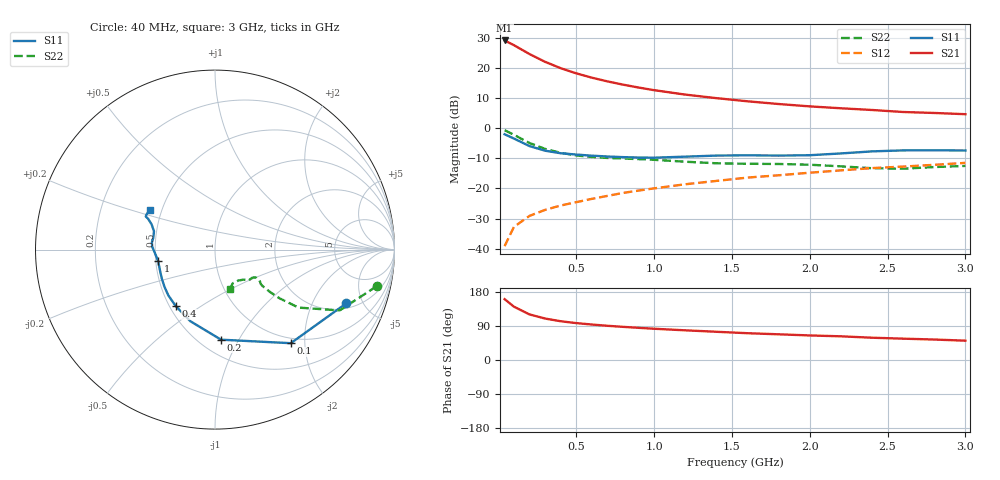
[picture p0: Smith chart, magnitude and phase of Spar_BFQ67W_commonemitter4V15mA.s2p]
! Filename:  BFQ67WD.S2P  Version:  4.0
! NXP part #: BFQ67W  Date: Jun 1994
! Bias condition: Vce=4V, Ic=15mA
#  MHz  S  MA  R  50
! Freq  S11  S21  S12  S22  !GUM [dB]
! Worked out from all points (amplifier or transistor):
!   21 points, 40 MHz to 3 GHz, reference 50 ohm
!   highest |S21| = 29.1 dB at 40 MHz (marker M1)
!   |S21| within 3 dB of that: start of sweep to 148.6 MHz
!   unconditionally stable (mu >= 1): 677.7 MHz to end of sweep
!   at 300 MHz: K = 0.73, MSG = 24.6 dB, |S12| = -27.1 dB
!   at 1 GHz: K = 1.07, MAG = 14.6 dB, |S12| = -20.0 dB
!   at 3 GHz: K = 1.01, MAG = 7.5 dB, |S12| = -11.5 dB
!   lowest NFmin = 1.95 dB at 1 GHz
!   S11 on the Smith chart (normalised r, x): 40 MHz: 2.32, -3.69; 100 MHz: 0.91, -1.72; 200 MHz: 0.63, -0.85; 400 MHz: 0.54, -0.40; 1 GHz: 0.52, -0.07; 3 GHz: 0.43, +0.23
40  0.79 -22.3  28.45 160.6  0.011 77.9  0.923 -12.8
100  0.671 -51.0  23.73 140.7  0.023 66.3  0.773 -26.0
200  0.503 -86.2  16.93 120.3  0.035 59.3  0.566 -34.8
300  0.422 -109.0  12.58 109.4  0.044 59.2  0.452 -37.0
400  0.383 -124.9  9.869 102.3  0.052 61.1  0.389 -37.6
500  0.364 -135.7  8.104 97.4  0.059 62.9  0.352 -37.6
600  0.349 -144.0  6.867 93.6  0.067 64.4  0.332 -37.4
700  0.338 -151.0  5.962 90.3  0.075 66.2  0.32 -37.0
800  0.33 -157.1  5.263 87.5  0.084 67.7  0.313 -36.1
900  0.325 -163.0  4.713 84.9  0.092 68.6  0.306 -35.2
1000  0.323 -168.5  4.261 82.5  0.1 69.3  0.298 -34.5
1200  0.336 -177.1  3.598 78.3  0.117 70.4  0.277 -34.2
1400  0.35 177.6  3.142 74.5  0.133 71.3  0.261 -36.6
1600  0.354 173.6  2.785 70.7  0.151 71.1  0.256 -40.7
1800  0.35 169.2  2.51 67.8  0.165 71.7  0.254 -43.0
2000  0.355 163.3  2.293 64.8  0.182 71.9  0.247 -43.9
2200  0.38 158.3  2.133 62.5  0.199 72.5  0.232 -46.0
2400  0.411 155.2  1.998 58.8  0.217 72.1  0.216 -53.0
2600  0.427 154.5  1.85 56.3  0.23 71.4  0.212 -62.0
2800  0.429 153.1  1.783 54.0  0.246 71.7  0.226 -67.3
3000  0.425 149.1  1.701 51.0  0.265 71.2  0.236 -69.8
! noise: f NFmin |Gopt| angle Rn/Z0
1000  1.95  0.2  100  0.251
